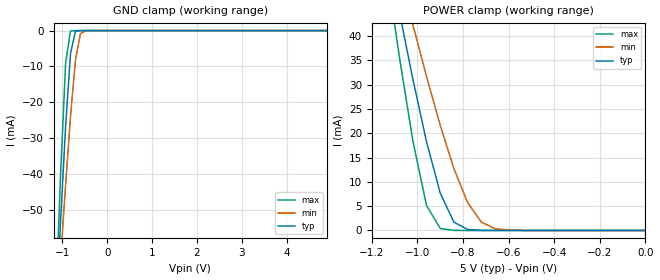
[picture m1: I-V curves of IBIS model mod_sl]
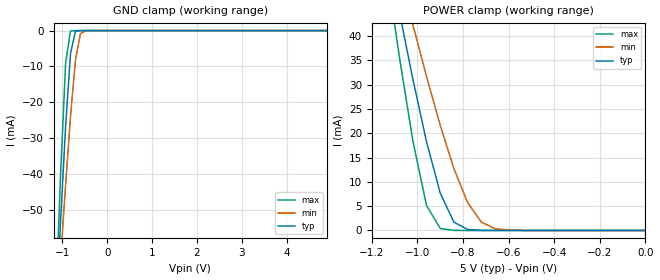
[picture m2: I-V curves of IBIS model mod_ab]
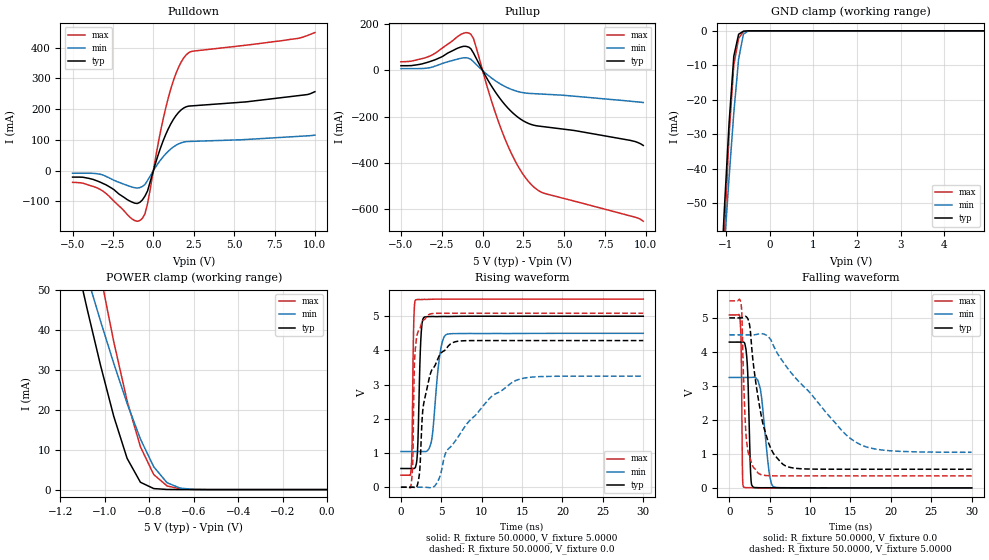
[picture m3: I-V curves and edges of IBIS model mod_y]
| IBIS (I/O, Buffer, Information, Specification) Model, officially
| electronic behavioral standard for Buffer structures of digital pins.
[IBIS ver]  4.0
[File name] 54ac157_5v0_rev1.ibs
[File Rev]  1.0
[Date]   19 Sep 2018
[Source]   CAD & Design Services (Catania) - STMicroelectronics
[Notes]
  (Note1) This IBIS model is the model of the product with package
   (Flat16 package elements);
  (Note2) This IBIS model is extracted with nominal 5.0V power supply
   (min:4.5V, typ:5.0V, max:5.5V);
  (Note3) This model has few Warnings about the non-monotonicity
   of I-V curves, but they are not indicative of problems
   inside the model;
[Copyright] (c) 2018 STMicroelectronics
|   Component RHF54AC157
[Component] RHF54AC157
[Manufacturer] STMicroelectronics
[Package]
| variable   typ   min   max
R_pkg   0.0   0.0   0.0
L_pkg   0.0H   0.0H   0.0H
C_pkg   0.0F   0.0F   0.0F
[Pin]   signal_name   model_name   R_pin   L_pin   C_pin
1   SELECT   mod_sl   87.8m   2.68nH   1.16pF
2   1A   mod_ab   53.6m   1.94nH   1.11pF
3   1B   mod_ab   34.1m   1.02nH   0.87pF
4   1Y   mod_y   34.1m   1.02nH   0.87pF
5   2A   mod_ab   34.1m   1.02nH   0.87pF
6   2B   mod_ab   34.1m   1.02nH   0.87pF
7   2Y   mod_y   53.6m   1.94nH   1.11pF
8   GND   GND   87.8m   2.68nH   1.16pF
9   3Y   mod_y   87.8m   2.68nH   1.16pF
10   3B   mod_ab   53.6m   1.94nH   1.11pF
11   3A   mod_ab   34.1m   1.02nH   0.87pF
12   4Y   mod_y   34.1m   1.02nH   0.87pF
13   4B   mod_ab   34.1m   1.02nH   0.87pF
14   4A   mod_ab   34.1m   1.02nH   0.87pF
15   STROB   mod_sl   53.6m   1.94nH   1.11pF
16   VCC   POWER   87.8m   2.68nH   1.16pF
| Models and submodels in the file (3): mod_sl (Input), mod_ab (Input), mod_y (I/O)
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|   Model mod_sl
[Model]   mod_sl
Model_type Input
Vinl   =   0.800V
Vinh   =   2.000V
C_comp   0.485pF   0.443pF   0.532pF
[Temperature Range]   25.0000   0.1250k   -55.0000
[Voltage Range]   5.0000V   4.5000V   5.5000V
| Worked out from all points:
|   GND clamp passes 1 mA (typ) near -0.72 V on its own axis
|   POWER clamp passes 1 mA (typ) near -0.81 V on its own axis
[GND_clamp]
|Voltage   I(typ)   I(min)   I(max)
-5V       -1.137A    -890.6mA   -1.482A
-1.15V    -80.1mA    -84.89mA   -75.58mA
-1.04V    -52.41mA   -63.51mA   -39.36mA
-930mV    -26.56mA   -42.88mA   -8.945mA
-820mV    -6.247mA   -23.72mA   -92.58uA
-710mV    -202uA     -8.108mA   -269.9nA
-600mV    -2.872uA   -885.3uA   -789.3pA
-490mV    -39.72nA   -40.33uA   -15.19pA
4.9V      9.6pA      196.2nA    8.6pA
[POWER_clamp]
|Voltage   I(typ)   I(min)   I(max)
-4.98V    1.112A     866.7mA    1.456A
-1.14V    59.95mA    64.87mA    55.2mA
-1.08V    45.21mA    53.46mA    35.95mA
-1.02V    31.13mA    42.35mA    18.39mA
-960mV    18.22mA    31.66mA    5.111mA
-900mV    7.676mA    21.64mA    415uA
-840mV    1.713mA    12.72mA    18.08uA
-780mV    205.2uA    5.745mA    745.1nA
-720mV    20.39uA    1.734mA    30.64nA
-660mV    1.979uA    364.6uA    1.272nA
-600mV    191.5nA    66.12uA    65.13pA
0V        10pA       55.89pA    11pA
|   Model mod_ab
[Model]   mod_ab
Model_type Input
Vinl   =   0.800V
Vinh   =   2.000V
C_comp   0.508pF   0.386pF   0.670pF
[Temperature Range]   25.0000   0.1250k   -55.0000
[Voltage Range]   5.0000V   4.5000V   5.5000V
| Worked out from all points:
|   GND clamp passes 1 mA (typ) near -0.72 V on its own axis
|   POWER clamp passes 1 mA (typ) near -0.81 V on its own axis
[GND_clamp]
|Voltage   I(typ)   I(min)   I(max)
-5V       -1.137A    -890.6mA   -1.482A
-1.15V    -80.1mA    -84.89mA   -75.58mA
-1.04V    -52.41mA   -63.51mA   -39.36mA
-930mV    -26.56mA   -42.88mA   -8.945mA
-820mV    -6.247mA   -23.72mA   -92.58uA
-710mV    -202uA     -8.108mA   -269.9nA
-600mV    -2.872uA   -885.3uA   -789.3pA
-490mV    -39.72nA   -40.33uA   -15.19pA
4.9V      9.6pA      196.2nA    8.6pA
[POWER_clamp]
|Voltage   I(typ)   I(min)   I(max)
-4.98V    1.112A     866.7mA    1.456A
-1.14V    59.95mA    64.87mA    55.2mA
-1.08V    45.21mA    53.46mA    35.95mA
-1.02V    31.13mA    42.35mA    18.39mA
-960mV    18.22mA    31.66mA    5.111mA
-900mV    7.676mA    21.64mA    415uA
-840mV    1.713mA    12.72mA    18.08uA
-780mV    205.2uA    5.745mA    745.1nA
-720mV    20.39uA    1.734mA    30.64nA
-660mV    1.979uA    364.6uA    1.272nA
-600mV    191.5nA    66.12uA    65.13pA
0V        10pA       55.89pA    11pA
|   Model mod_y
[Model]   mod_y
Model_type I/O
Polarity   Non-Inverting
Vinl   =  0.800V
Vinh   =  2.000V
Vmeas   =  2.500V
Cref   =  50pF
Rref   =  500
C_comp   2.952pF   2.119pF   3.856pF
[Temperature Range]  25.0000   0.1250k   -55.0000
[Voltage Range]   5.0000V   4.5000V   5.5000V
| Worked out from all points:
|   slope of the pulldown table from 0 to 0.75 V, typ, clamps not added: 6.47 ohm
|   slope of the pullup table from 0 to 0.75 V, typ, clamps not added: 8.35 ohm
|   GND clamp passes 1 mA (typ) near -0.71 V on its own axis
|   POWER clamp passes 1 mA (typ) near -0.81 V on its own axis
|   rising waveform, R_fixture 50.0000, V_fixture 5.0000: 20-80 % time 307ps typ, 798ps min, 166ps max; typ from 0.548 V to 5 V
|   rising waveform, R_fixture 50.0000, V_fixture 0.0: 20-80 % time 1.42ns typ, 5.83ns min, 303ps max; typ from 0 V to 4.29 V
|   falling waveform, R_fixture 50.0000, V_fixture 0.0: 20-80 % time 308ps typ, 810ps min, 135ps max; typ from 4.29 V to 0 V
|   falling waveform, R_fixture 50.0000, V_fixture 5.0000: 20-80 % time 1.92ns typ, 7.39ns min, 510ps max; typ from 5 V to 0.548 V
[Pulldown]
|Voltage   I(typ)   I(min)   I(max)
-5V       -20.74mA   -8.151mA   -37.83mA
-3.24V    -38.35mA   -12.05mA   -62.33mA
-1.32V    -102mA     -53.16mA   -157mA
-840mV    -103mA     -55.05mA   -162.2mA
-520mV    -82.67mA   -45.04mA   -140.4mA
-360mV    -65.93mA   -31.71mA   -107.9mA
440mV     73.46mA    34.38mA    126.4mA
1.08V     152.3mA    70.68mA    266mA
1.56V     189.5mA    87.25mA    336.3mA
2.04V     208.1mA    94.66mA    377.2mA
8.92V     243.8mA    111.5mA    430.1mA
10V       257mA      115.7mA    449.3mA
[Pullup]
|Voltage   I(typ)   I(min)   I(max)
-5V       20.74mA    8.151mA    37.83mA
-3.24V    38.35mA    12.05mA    62.33mA
-1.32V    102mA      53.16mA    157mA
-720mV    94.48mA    48.73mA    157.2mA
-560mV    76.12mA    38.03mA    139.1mA
560mV     -69.07mA   -33.2mA    -135.3mA
1.36V     -147.6mA   -69.01mA   -294.6mA
2.16V     -202.5mA   -91.16mA   -413.9mA
2.96V     -233.7mA   -99.72mA   -493.1mA
3.76V     -243.9mA   -102.8mA   -532.4mA
9.04V     -303mA     -133.1mA   -630.6mA
9.84V     -325mA     -138.8mA   -654mA
[GND_clamp]
|Voltage   I(typ)   I(min)   I(max)
-5V       -1.137A    -890.6mA   -1.489A
-1.15V    -80.38mA   -84.94mA   -95.23mA
-1.04V    -52.79mA   -63.56mA   -60.94mA
-930mV    -27.16mA   -42.95mA   -30.74mA
-820mV    -7.378mA   -23.82mA   -9.928mA
-710mV    -1.011mA   -8.232mA   -2.205mA
-600mV    -110.5uA   -965.7uA   -202.6uA
-490mV    -9.509uA   -58.07uA   -7.181uA
-380mV    -722.2nA   -4.418uA   -236.7nA
4.9V      105.2pA    213.3nA    21.77pA
[POWER_clamp]
|Voltage   I(typ)   I(min)   I(max)
-4.98V    1.112A     866.7mA    1.476A
-1.14V    60.04mA    64.85mA    90.87mA
-1.08V    45.32mA    53.44mA    71.97mA
-1.02V    31.25mA    42.32mA    53.89mA
-960mV    18.36mA    31.63mA    37.06mA
-900mV    7.838mA    21.6mA     22.26mA
-840mV    1.841mA    12.69mA    10.74mA
-780mV    258.7uA    5.713mA    3.765mA
-720mV    36.78uA    1.715mA    918.5uA
-660mV    6.646uA    359.7uA    189.7uA
-600mV    1.494uA    65.41uA    37.7uA
0V        111.1pA    2.989nA    31.8pA
[Ramp]
| variable   typ   min   max
dV/dt_r   2.5730/1.4663n   1.9492/5.8177n   3.0520/0.3798n
dV/dt_f   2.6712/1.9081n   2.0731/7.3425n   3.0890/0.5652n
R_load = 50.0000
[Rising Waveform]
R_fixture= 50.0000
V_fixture= 5.0000
V_fixture_min= 4.5000
V_fixture_max= 5.5000
|time   V(typ)   V(min)   V(max)
0s        547.7mV    1.045V     351.6mV
1.26ns    547.7mV    1.045V     510.9mV
1.38ns    547.9mV    1.045V     1.255V
1.56ns    546.3mV    1.045V     4.572V
1.8ns     584.4mV    1.045V     5.475V
2.1ns     1.31V      1.045V     5.489V
2.46ns    4.316V     1.045V     5.487V
2.82ns    4.961V     1.044V     5.492V
5.64ns    4.992V     4.469V     5.5V
30ns      5V         4.5V       5.5V
[Rising Waveform]
R_fixture= 50.0000
V_fixture= 0.0
V_fixture_min= 0.0
V_fixture_max= 0.0
|time   V(typ)   V(min)   V(max)
0s        0V         0V         0V
1.26ns    -14.36uV   -1.065uV   71.85mV
1.47ns    731.3uV    -4.228uV   792.4mV
1.62ns    -4.62mV    -1.918uV   3.14V
1.8ns     -18.01mV   -896nV     4.09V
2.28ns    377.5mV    -6.094uV   4.608V
3.36ns    3.035V     -7.485mV   5.035V
6.42ns    4.229V     1.255V     5.087V
14.22ns   4.288V     3.122V     5.087V
30ns      4.288V     3.248V     5.087V
[Falling Waveform]
R_fixture= 50.0000
V_fixture= 0.0
V_fixture_min= 0.0
V_fixture_max= 0.0
|time   V(typ)   V(min)   V(max)
0s        4.288V     3.248V     5.087V
1.38ns    4.288V     3.248V     4.803V
1.5ns     4.289V     3.248V     3.601V
1.62ns    4.292V     3.248V     617.8mV
1.74ns    4.291V     3.248V     29.02mV
2.22ns    3.652V     3.248V     5.517mV
2.64ns    426.7mV    3.25V      5.641mV
2.97ns    14.69mV    3.253V     3.83mV
5.52ns    2.457mV    27.44mV    195.4uV
30ns      -53.84nV   8.747uV    -322.6nV
[Falling Waveform]
R_fixture= 50.0000
V_fixture= 5.0000
V_fixture_min= 4.5000
V_fixture_max= 5.5000
|time   V(typ)   V(min)   V(max)
0s        5V         4.5V       5.5V
1.44ns    5V         4.5V       5.435V
1.56ns    5V         4.5V       5.074V
2.1ns     5.034V     4.5V       1.457V
2.52ns    4.78V      4.5V       897mV
3.66ns    2.518V     4.529V     419.9mV
5.16ns    1.146V     4.349V     355.5mV
7.26ns    619.1mV    3.505V     351.7mV
16.47ns   547.7mV    1.244V     351.6mV
30ns      547.7mV    1.046V     351.6mV
